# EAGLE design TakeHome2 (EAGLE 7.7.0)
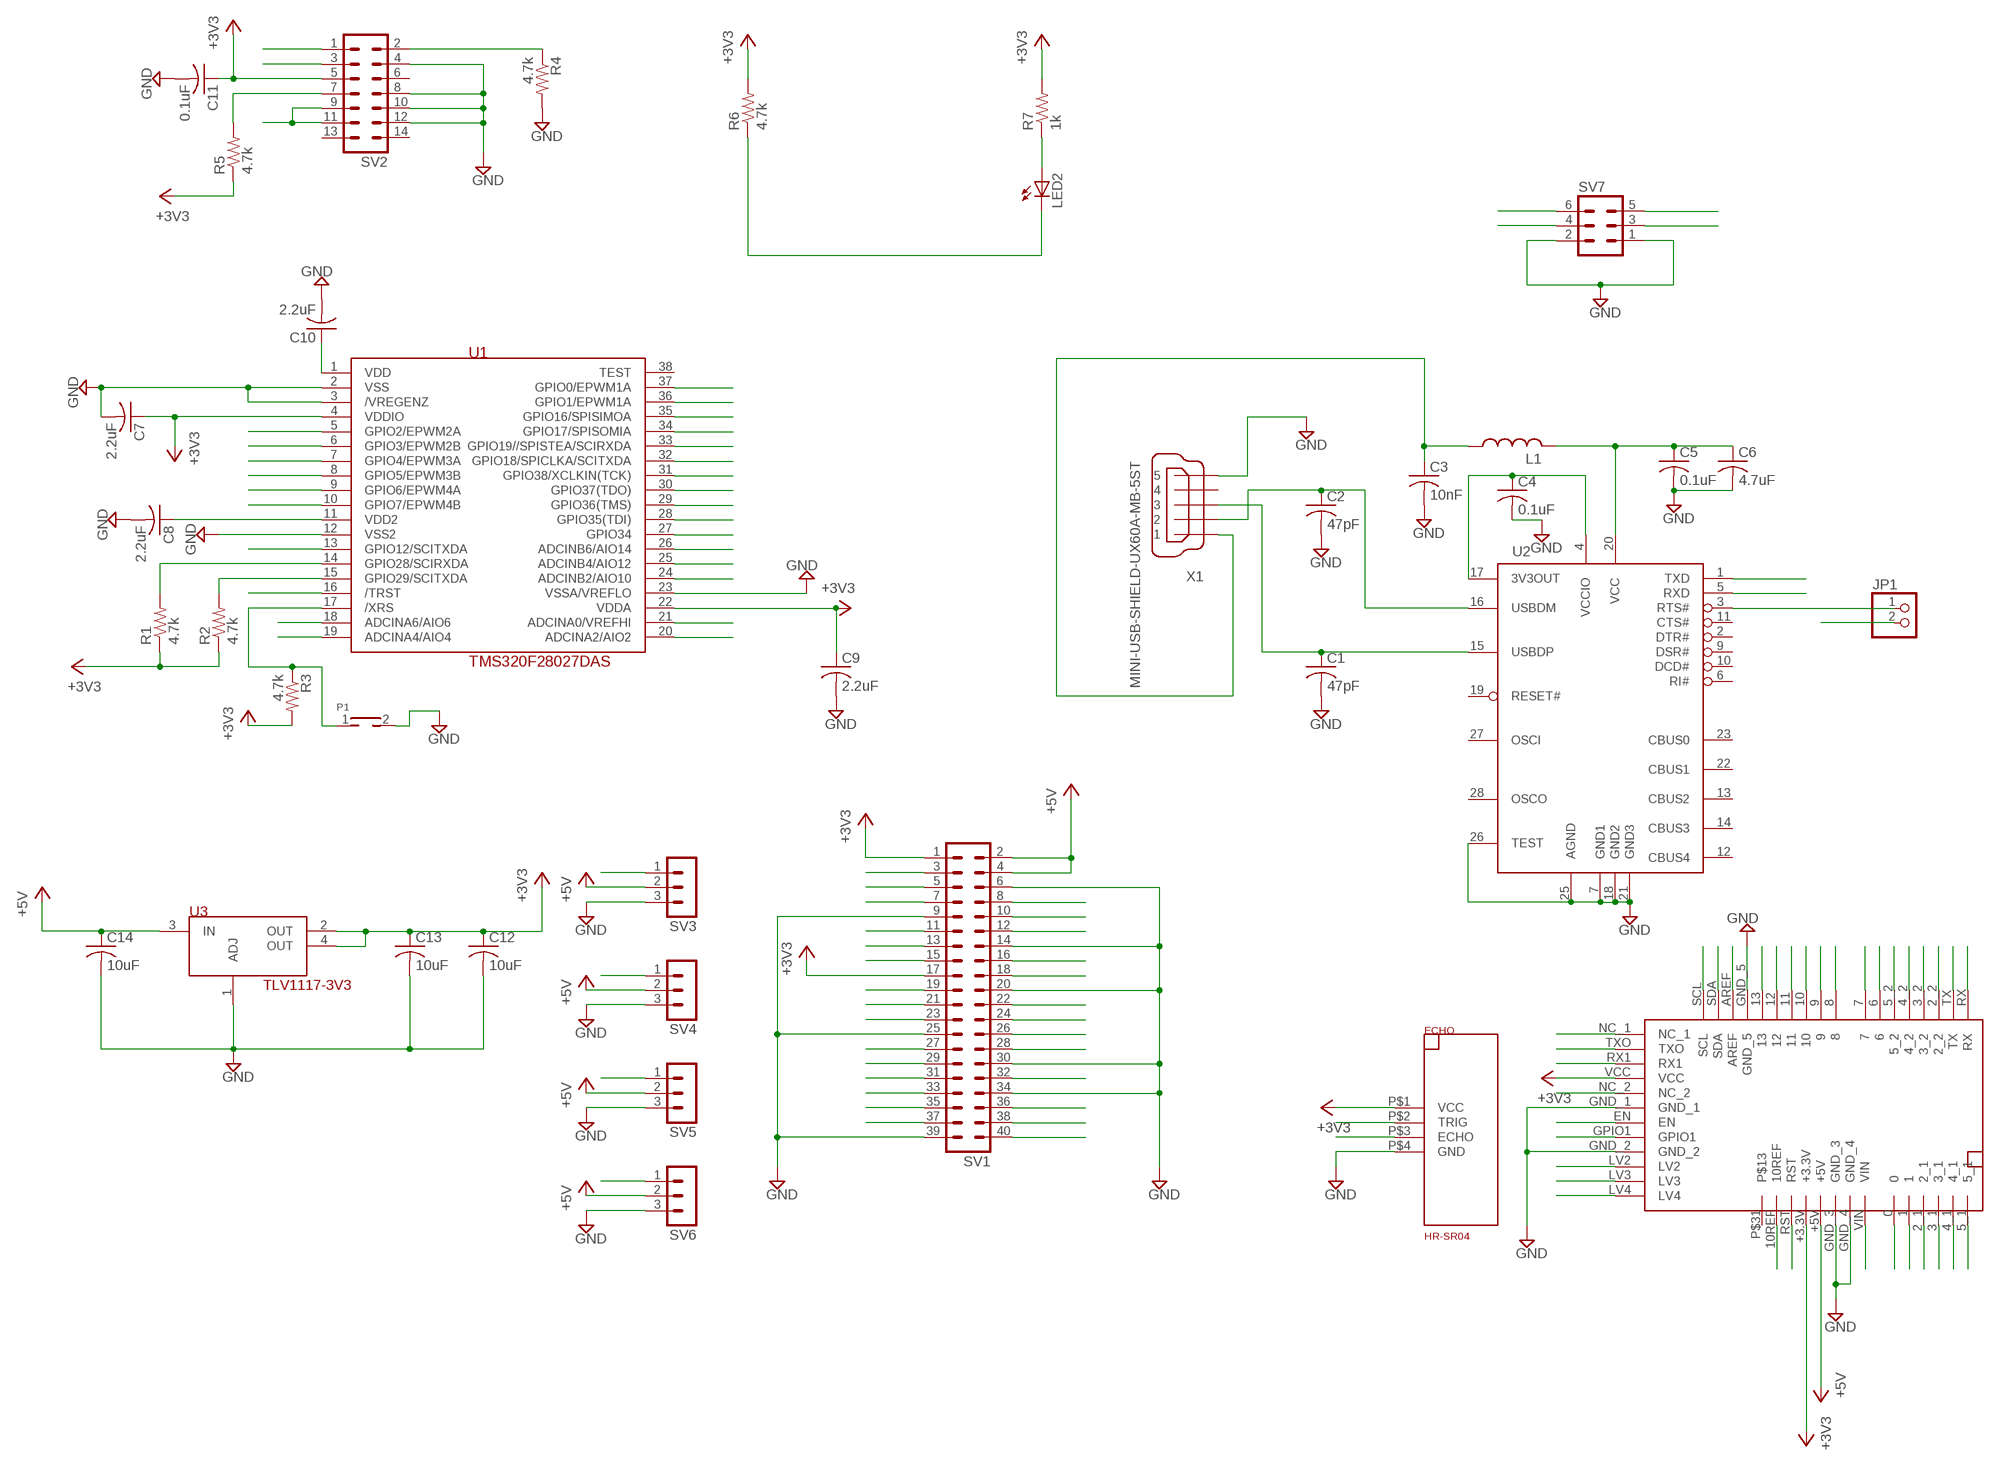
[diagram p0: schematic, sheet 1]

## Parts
C1  47pF  C-US025-025X050  [C025-025X050]
C2  47pF  C-US025-025X050  [C025-025X050]
C3  10nF  C-US025-025X050  [C025-025X050]
C4  0.1uF  C-US025-025X050  [C025-025X050]
C5  0.1uF  C-US025-025X050  [C025-025X050]
C6  4.7uF  C-US025-025X050  [C025-025X050]
C7  2.2uF  C-US025-025X050  [C025-025X050]
C8  2.2uF  C-US025-025X050  [C025-025X050]
C9  2.2uF  C-US025-025X050  [C025-025X050]
C10  2.2uF  C-US025-025X050  [C025-025X050]
C11  0.1uF  C-US025-025X050  [C025-025X050]
C12  10uF  C-US025-025X050  [C025-025X050]
C13  10uF  C-US025-025X050  [C025-025X050]
C14  10uF  C-US025-025X050  [C025-025X050]
ECHO  HR-SR04  [HC-SR04]
JP1  PINHD-1X2  [1X02]
L1  L-US0204/7  [0204/7]
LED2  LED5MM  [LED5MM]
P1  TH_PUSHBOTTON  [TH_PUSHBUTTON]
R1  4.7k  R-US_0204/5  [0204/5]
R2  4.7k  R-US_0204/5  [0204/5]
R3  4.7k  R-US_0204/5  [0204/5]
R4  4.7k  R-US_0204/5  [0204/5]
R5  4.7k  R-US_0204/5  [0204/5]
R6  4.7k  R-US_0204/5  [0204/5]
R7  1k  R-US_0204/5  [0204/5]
SV1  MA20-2  [MA20-2]
SV2  MA07-2  [MA07-2]
SV3  MA03-1  [MA03-1]
SV4  MA03-1  [MA03-1]
SV5  MA03-1  [MA03-1]
SV6  MA03-1  [MA03-1]
SV7  MA03-2  [MA03-2]
U1  TMS320F28027DAS  [DA38]
U2  FT232RL  [SSOP28DB]
U3  TLV1117-3V3  [SOT223]
U$1  M6E_NANO  [M6E_NANO]
X1  MINI-USB-SHIELD-UX60A-MB-5ST  [UX60A-MB-5ST]

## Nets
0: U$1.0
1: U$1.1
2: U$1.2_1 U$1.2_2
3: U$1.3_1 U$1.3_2
4: U$1.4_1 U$1.4_2
5: U$1.5_1 U$1.5_2
6: U$1.6
7: U$1.7
8: U$1.8
9: U$1.9
10: U$1.10
10REF: U$1.10REF
11: U$1.11
12: U$1.12
13: U$1.13
+3V3 [supply]: C7.1 C9.1 C11.1 C12.1 C13.1 ECHO.P$1(VCC) R1.1 R2.1 R3.2 R5.1 R6.2 R7.2 SV1.1 SV1.17 SV2.5 U1.4(VDDIO) U1.22(VDDA) U3.2(OUT) U3.4(OUT) U$1.+3.3V U$1.VCC
+5V [supply]: C14.1 SV1.2 SV1.4 SV3.2 SV4.2 SV5.2 SV6.2 U3.3(IN) U$1.+5V
/SPISTEA: SV1.24 U1.33(GPIO19//SPISTEA/SCIRXDA)
ADCA0: SV1.27 U1.21(ADCINA0/VREFHI)
ADCA2: SV1.29 U1.20(ADCINA2/AIO2)
ADCA4: SV1.31 U1.19(ADCINA4/AIO4)
ADCA6: SV1.33 U1.18(ADCINA6/AIO6)
ADCB2: SV1.26 U1.24(ADCINB2/AIO10)
ADCB4: SV1.28 U1.25(ADCINB4/AIO12)
ADCB6: SV1.32 U1.26(ADCINB6/AIO14)
AREF: U$1.AREF
ECHO: ECHO.P$3(ECHO)
EN: U$1.EN
GND [supply]: C1.2 C2.2 C3.2 C4.2 C5.2 C6.2 C7.2 C8.2 C9.2 C10.2 C11.2 C12.2 C13.2 C14.2 ECHO.P$4(GND) P1.2 R4.2 SV1.6 SV1.9 SV1.14 SV1.20 SV1.25 SV1.30 SV1.34 SV1.39 SV2.4 SV2.8 SV2.10 SV2.12 SV3.3 SV4.3 SV5.3 SV6.3 SV7.1 SV7.2 U1.2(VSS) U1.3(/VREGENZ) U1.12(VSS2) U1.23(VSSA/VREFLO) U2.7(GND1) U2.18(GND2) U2.21(GND3) U2.25(AGND) U2.26(TEST) U3.1(ADJ) U$1.GND_1 U$1.GND_2 U$1.GND_3 U$1.GND_4 U$1.GND_5 X1.5
GPIO0: SV1.7 U1.37(GPIO0/EPWM1A)
GPIO1: SV1.11 U1.36(GPIO1/EPWM1A) U$1.GPIO1
GPIO2: SV1.13 SV3.1 U1.5(GPIO2/EPWM2A)
GPIO3: SV1.15 SV4.1 U1.6(GPIO3/EPWM2B)
GPIO4: SV1.12 SV5.1 U1.7(GPIO4/EPWM3A)
GPIO5: SV1.16 SV6.1 U1.8(GPIO5/EPWM3B)
GPIO6: SV1.18 U1.9(GPIO6/EPWM4A)
GPIO7: SV1.38 U1.10(GPIO7/EPWM4B)
GPIO12: SV1.36 U1.13(GPIO12/SCITXDA)
GPIO34: LED2.K(C) R6.1 SV1.22 U1.27(GPIO34)
LV2: U$1.LV2
LV3: U$1.LV3
LV4: U$1.LV4
N$1: C5.1 C6.1 L1.2 U2.20(VCC)
N$2: C4.1 U2.4(VCCIO) U2.17(3V3OUT)
N$3: C3.1 L1.1 X1.1
N$4: C2.1 U2.16(USBDM) X1.2
N$5: C1.1 U2.15(USBDP) X1.3
N$6: LED2.A R7.1
N$7: C8.1 U1.11(VDD2)
N$8: P1.1 R3.1 U1.17(/XRS)
N$10: C10.1 U1.1(VDD)
N$38: U$1.TX
N$39: U$1.RX
NC: U$1.NC_1 U$1.NC_2
RST: U$1.RST
RTS_FT232RL: JP1.1 U2.3(RTS#)
RX1: U$1.RX1
RXD_FT232RL: SV7.3 U2.5(RXD)
SCL: R2.2 SV1.5 SV1.8 SV7.4 U1.15(GPIO29/SCITXDA) U$1.SCL
SDA: R1.2 SV1.3 SV1.10 SV7.6 U1.14(GPIO28/SCIRXDA) U$1.SDA
SPICLKA: SV1.23 U1.32(GPIO18/SPICLKA/SCITXDA)
SPISIMOA: SV1.19 U1.35(GPIO16/SPISIMOA)
SPISOMIA: SV1.21 U1.34(GPIO17/SPISOMIA)
TCK: SV1.40 SV2.9 SV2.11 U1.31(GPIO38/XCLKIN(TCK))
TDI: SV1.35 SV2.3 U1.28(GPIO35(TDI))
TDO: JP1.2 R5.2 SV2.7 U1.30(GPIO37(TDO))
TMS: SV1.37 SV2.1 U1.29(GPIO36(TMS))
TRIG: ECHO.P$2(TRIG)
TRSTN: R4.1 SV2.2 U1.16(/TRST)
TXD_FT232RL: SV7.5 U2.1(TXD)
TXO: U$1.TXO
VIN: U$1.VIN
Unconnected: SV2.6 SV2.13 SV2.14 U1.38(TEST) U2.2(DTR#) U2.6(RI#) U2.9(DSR#) U2.10(DCD#) U2.11(CTS#) U2.12(CBUS4) U2.13(CBUS2) U2.14(CBUS3) U2.19(RESET#) U2.22(CBUS1) U2.23(CBUS0) U2.27(OSCI) U2.28(OSCO) U$1.P$31 X1.4 X1.M1(S1) X1.M2(S2) X1.M3(S3) X1.M4(S4)

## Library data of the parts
C1-C14 = rcl:C-US: CAPACITOR, American symbol
ECHO = SE423EagleLibrary:HR-SR04
JP1 = pinhead:PINHD-1X2: PIN HEADER
L1 = rcl:L-US: INDUCTOR, American symbol
LED2 = led:LED: LED
P1 = SE423EagleLibrary:TH_PUSHBOTTON
R1-R7 = rcl:R-US_: RESISTOR, American symbol
SV1 = con-lstb:MA20-2: PIN HEADER; OC_FARNELL: unknown; OC_NEWARK: unknown
SV2 = con-lstb:MA07-2: PIN HEADER; OC_FARNELL: unknown; OC_NEWARK: unknown
SV3-SV6 = con-lstb:MA03-1: PIN HEADER; OC_FARNELL: unknown; OC_NEWARK: unknown
SV7 = con-lstb:MA03-2: PIN HEADER; OC_FARNELL: unknown; OC_NEWARK: unknown
U1 = SE423EagleLibrary:TMS320F28027DAS
U2 = SE423EagleLibrary:FT232RL: USB UART 4th Generation USB UART (USB <-> Serial) Controller
U3 = SE423EagleLibrary:TLV1117-3V3
U$1 = SE423EagleLibrary:M6E_NANO
X1 = SE423EagleLibrary:MINI-USB-SHIELD-: MINI USB Connector Source: http://www.hirose.co.jp/cataloge_hp/e24000019.pdf; OC_FARNELL: unknown; OC_NEWARK: unknown

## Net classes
0 default: width 0.203 mm, drill 0.508 mm, clearance 0.203 mm
1 supply: width 0.508 mm, drill 0.508 mm, clearance 0.203 mm

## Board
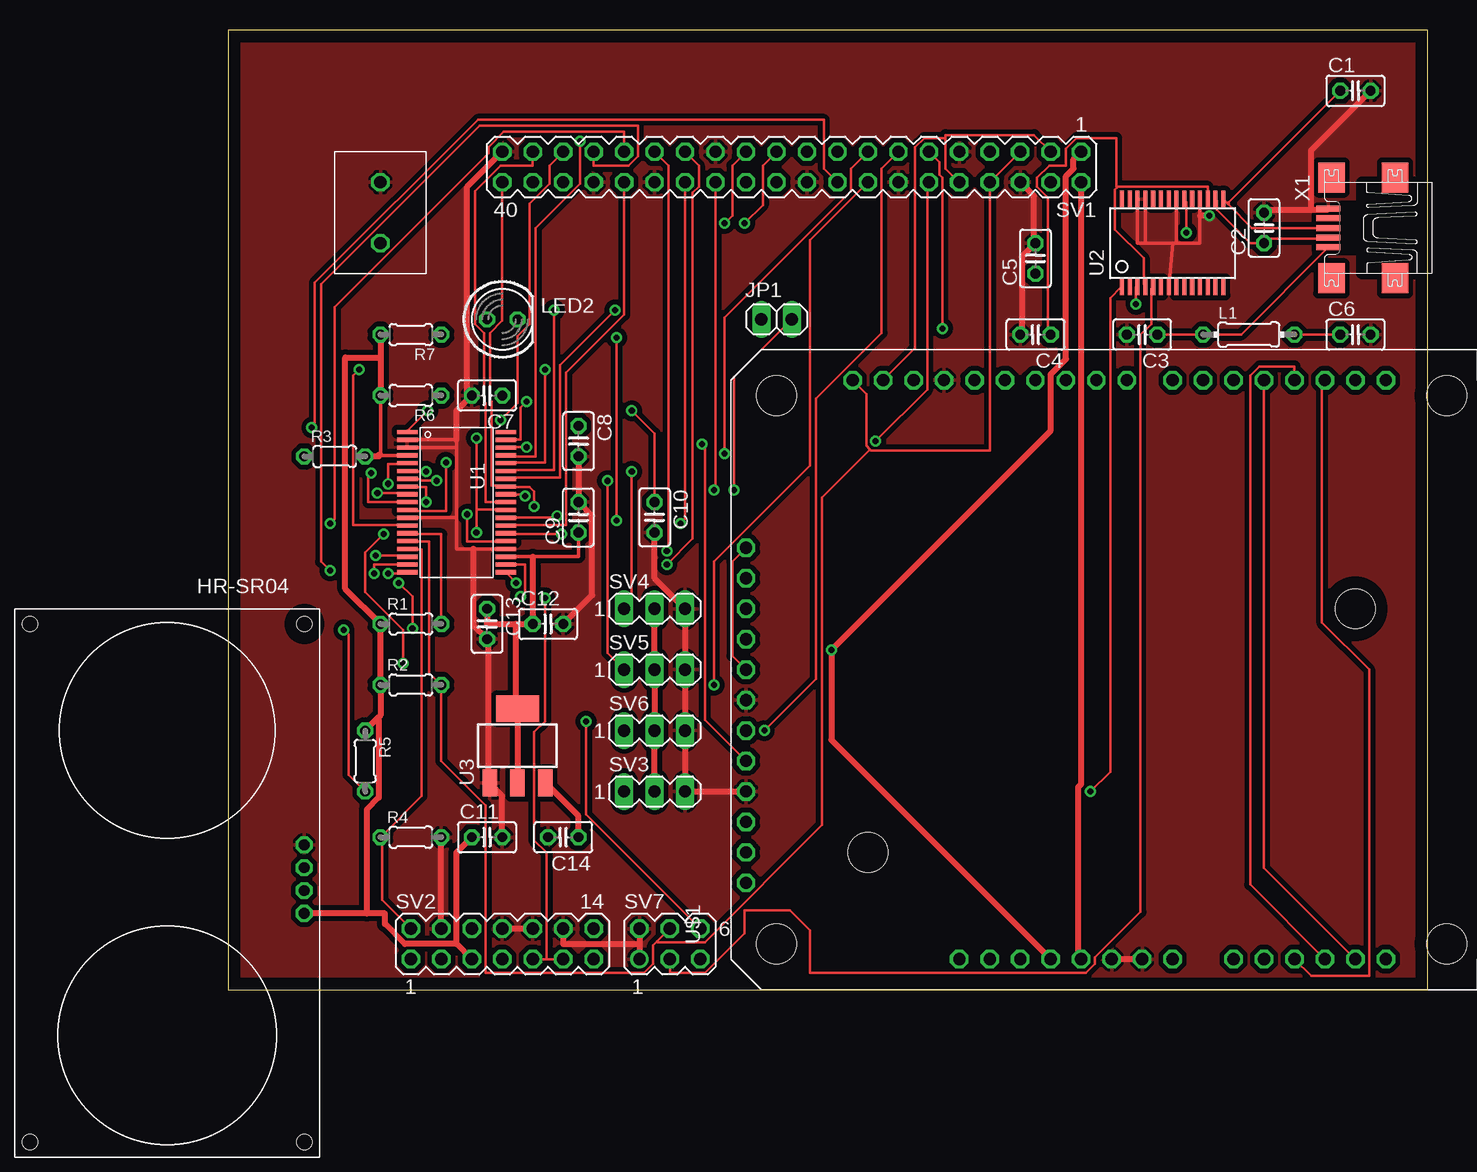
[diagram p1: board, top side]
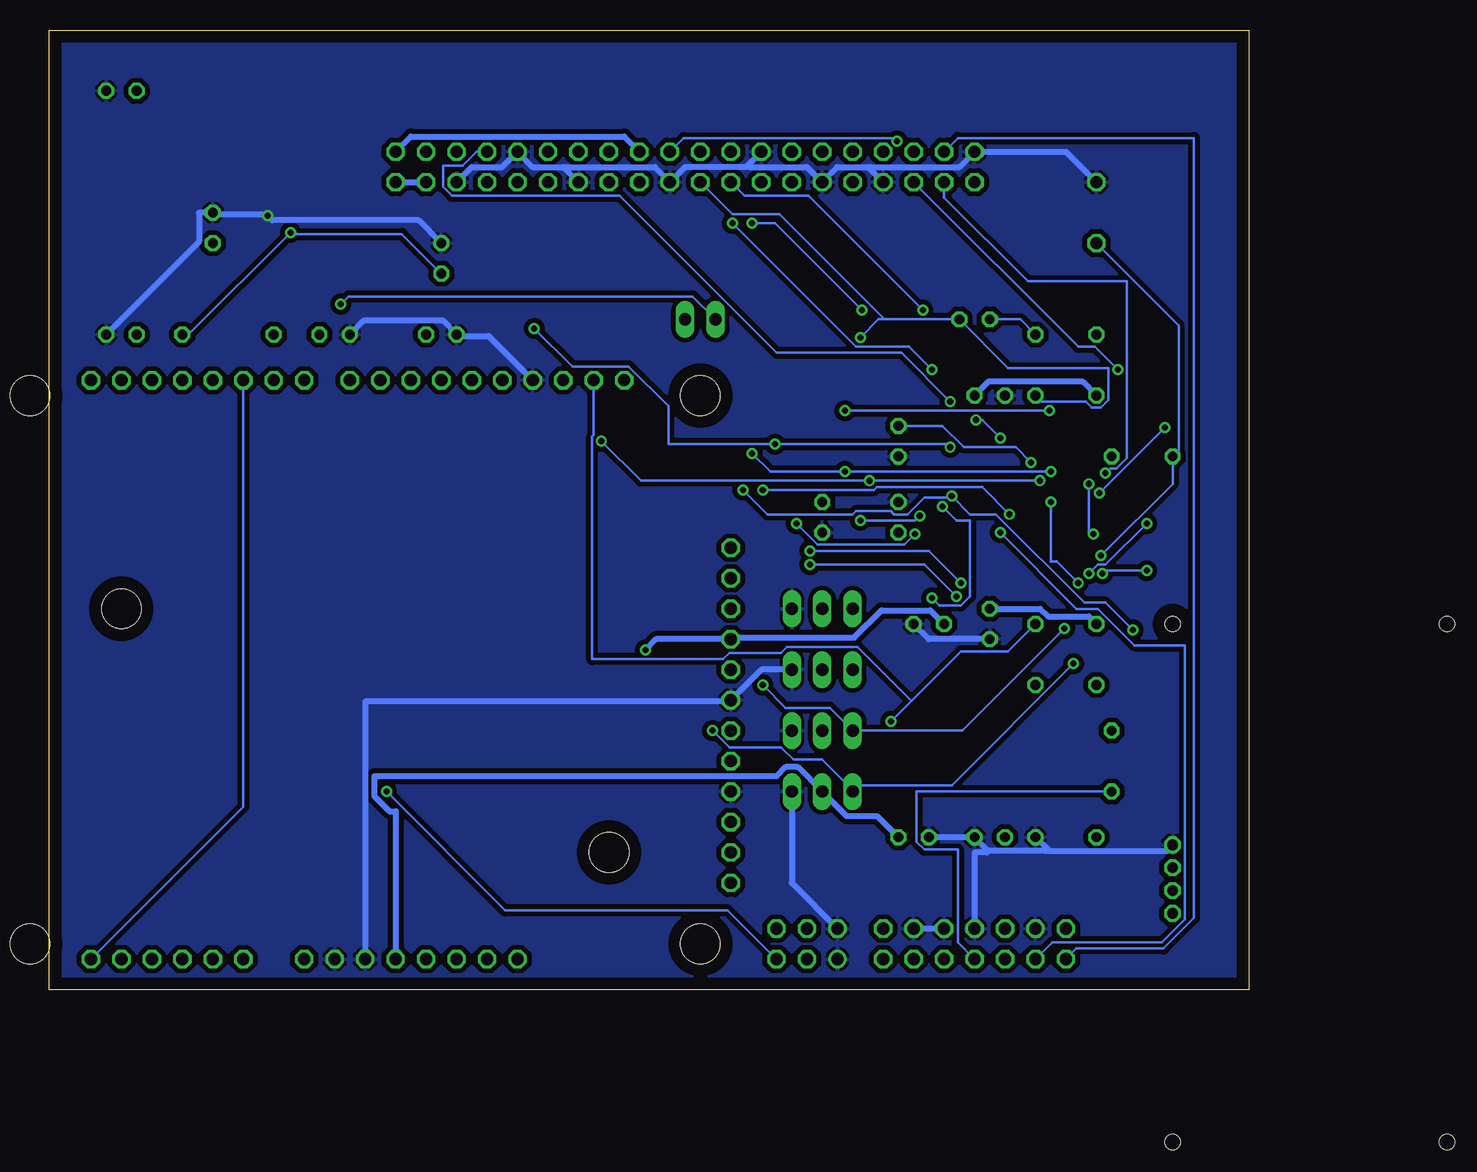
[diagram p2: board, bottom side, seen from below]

Size 100 x 80 mm. Coordinates in mm from the lower left corner, seen from the top.
Outline: 0,0 100,0 100,80 0,80 0,0
Copper layers (1*16): Top 0.035mm / dielectric 1.5mm / Bottom 0.035mm
Design rules "default *": minimum track width 8mil, minimum drill 20mil, track to track 8mil, track to pad 8mil, pad to pad 8mil, via to via 8mil, smd to smd 8mil, copper to edge 40mil, drill to drill 8mil, minimum pad ring 10mil, minimum via ring 8mil, stop-mask expansion 4mil, vias tented up to drill 20mil, thermal gap 10mil

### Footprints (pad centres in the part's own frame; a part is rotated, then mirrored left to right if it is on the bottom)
C025-025X050 = drill 0.813 octagon: 1 -1.27,0; 2 1.27,0
HC-SR04 = drill 0.889 octagon: P$1 1.27,25.4; P$2 1.27,23.495; P$3 1.27,21.59; P$4 1.27,19.685 | hole 1.27: 1.27,1.27; 1.27,44.45; 24.13,44.45; 24.13,1.27
1X02 = drill 1.016 long: 1 -1.27,0; 2 1.27,0
0204/7 = drill 0.813 octagon: 1 -3.81,0; 2 3.81,0
LED5MM = drill 0.813 octagon: A -1.27,0; K 1.27,0
TH_PUSHBUTTON = drill 1.016 octagon: 1 0,2.54; 2 0,-2.54
0204/5 = drill 0.813 octagon: 1 -2.54,0; 2 2.54,0
MA20-2 = drill 1.016 octagon: 1 -24.13,-1.27; 2 -24.13,1.27; 3 -21.59,-1.27; 4 -21.59,1.27; 5 -19.05,-1.27; 6 -19.05,1.27; 7 -16.51,-1.27; 8 -16.51,1.27; 9 -13.97,-1.27; 10 -13.97,1.27; 11 -11.43,-1.27; 12 -11.43,1.27; 13 -8.89,-1.27; 14 -8.89,1.27; 15 -6.35,-1.27; 16 -6.35,1.27; 17 -3.81,-1.27; 18 -3.81,1.27; 19 -1.27,-1.27; 20 -1.27,1.27; 21 1.27,-1.27; 22 1.27,1.27; 23 3.81,-1.27; 24 3.81,1.27; 25 6.35,-1.27; 26 6.35,1.27; 27 8.89,-1.27; 28 8.89,1.27; 29 11.43,-1.27; 30 11.43,1.27; 31 13.97,-1.27; 32 13.97,1.27; 33 16.51,-1.27; 34 16.51,1.27; 35 19.05,-1.27; 36 19.05,1.27; 37 21.59,-1.27; 38 21.59,1.27; 39 24.13,-1.27; 40 24.13,1.27
MA07-2 = drill 1.016 octagon: 1 -7.62,-1.27; 2 -7.62,1.27; 3 -5.08,-1.27; 4 -5.08,1.27; 5 -2.54,-1.27; 6 -2.54,1.27; 7 0,-1.27; 8 0,1.27; 9 2.54,-1.27; 10 2.54,1.27; 11 5.08,-1.27; 12 5.08,1.27; 13 7.62,-1.27; 14 7.62,1.27
MA03-1 = drill 1.016 long: 1 -2.54,0; 2 0,0; 3 2.54,0
MA03-2 = drill 1.016: 1 -2.54,-1.27 | drill 1.016 octagon: 2 -2.54,1.27; 3 0,-1.27; 4 0,1.27; 5 2.54,-1.27; 6 2.54,1.27
DA38 = smd 0.35 x 1.705: 1 -5.85,-4.12; 2 -5.2,-4.12; 3 -4.55,-4.12; 4 -3.9,-4.12; 5 -3.25,-4.12; 6 -2.6,-4.12; 7 -1.95,-4.12; 8 -1.3,-4.12; 9 -0.65,-4.12; 10 0,-4.12; 11 0.65,-4.12; 12 1.3,-4.12; 13 1.95,-4.12; 14 2.6,-4.12; 15 3.25,-4.12; 16 3.9,-4.12; 17 4.55,-4.12; 18 5.2,-4.12; 19 5.85,-4.12; 20 5.85,4.12; 21 5.2,4.12; 22 4.55,4.12; 23 3.9,4.12; 24 3.25,4.12; 25 2.6,4.12; 26 1.95,4.12; 27 1.3,4.12; 28 0.65,4.12; 29 0,4.12; 30 -0.65,4.12; 31 -1.3,4.12; 32 -1.95,4.12; 33 -2.6,4.12; 34 -3.25,4.12; 35 -3.9,4.12; 36 -4.55,4.12; 37 -5.2,4.12; 38 -5.85,4.12
SSOP28DB = smd 0.348 x 1.397: 1 -4.225,-3.656; 2 -3.575,-3.656; 3 -2.925,-3.656; 4 -2.275,-3.656; 5 -1.625,-3.656; 6 -0.975,-3.656; 7 -0.325,-3.656; 8 0.325,-3.656; 9 0.975,-3.656; 10 1.625,-3.656; 11 2.275,-3.656; 12 2.925,-3.656; 13 3.575,-3.656; 14 4.225,-3.656; 15 4.225,3.656; 16 3.575,3.656; 17 2.925,3.656; 18 2.275,3.656; 19 1.625,3.656; 20 0.975,3.656; 21 0.325,3.656; 22 -0.325,3.656; 23 -0.975,3.656; 24 -1.625,3.656; 25 -2.275,3.656; 26 -2.925,3.656; 27 -3.575,3.656; 28 -4.225,3.656
SOT223 = smd 1.219 x 2.235: 1 -2.311,-3.099; 2 0,-3.099; 3 2.311,-3.099 | smd 3.6 x 2.2: 4 0,3.099
M6E_NANO = drill 1.016 octagon: 0 41.91,2.54; 1 44.45,2.54; 2_1 46.99,2.54; 2_2 49.53,50.8; 3_1 49.53,2.54; 3_2 46.99,50.8; 4_1 52.07,2.54; 4_2 44.45,50.8; 5_1 54.61,2.54; 5_2 41.91,50.8; 6 39.37,50.8; 7 36.83,50.8; 8 33.02,50.8; 9 30.48,50.8; 10 27.94,50.8; 10REF 21.59,2.54; 11 25.4,50.8; 12 22.86,50.8; 13 20.32,50.8; +3.3V 26.67,2.54; +5V 29.21,2.54; AREF 15.24,50.8; EN 1.27,21.59; GND_1 1.27,24.13; GND_2 1.27,16.51; GND_3 31.75,2.54; GND_4 34.29,2.54; GND_5 17.78,50.8; GPIO1 1.27,19.05; LV2 1.27,13.97; LV3 1.27,11.43; LV4 1.27,8.89; NC_1 1.27,36.83; NC_2 1.27,26.67; P$31 19.05,2.54; RST 24.13,2.54; RX 54.61,50.8; RX1 1.27,31.75; SCL 10.16,50.8; SDA 12.7,50.8; TX 52.07,50.8; TXO 1.27,34.29; VCC 1.27,29.21; VIN 36.83,2.54 | hole 3.302: 3.81,3.81; 11.43,11.43; 3.81,49.53; 59.69,49.53; 59.69,3.81; 52.07,31.75
UX60A-MB-5ST = smd 2 x 0.5: 1 2.25,1.6; 2 2.25,0.8; 3 2.25,0; 4 2.25,-0.8; 5 2.25,-1.6 | smd 2.2 x 2.5: M1 -3.3,-4.2; M2 -3.3,4.2; M3 2,4.2; M4 2,-4.2

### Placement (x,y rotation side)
C1  93.98,74.93 0 top
C2  86.36,63.5 90 top
C3  76.2,54.61 180 top
C4  67.31,54.61 180 top
C5  67.31,60.96 90 top
C6  93.98,54.61 0 top
C7  21.59,49.53 180 top
C8  29.21,45.72 270 top
C9  29.21,39.37 90 top
C10  35.56,39.37 270 top
C11  21.59,12.7 0 top
C12  26.67,30.48 0 top
C13  21.59,30.48 270 top
C14  27.94,12.7 180 top
ECHO  7.62,31.75 180 top
JP1  45.72,55.88 0 top
L1  85.09,54.61 0 top
LED2  22.86,55.88 0 top
P1  12.7,64.77 180 top
R1  15.24,30.48 0 top
R2  15.24,25.4 0 top
R3  8.89,44.45 0 top
R4  15.24,12.7 0 top
R5  11.43,19.05 270 top
R6  15.24,49.53 180 top
R7  15.24,54.61 180 top
SV1  46.99,68.58 180 top
SV2  22.86,3.81 0 top
SV3  35.56,16.51 0 top
SV4  35.56,31.75 0 top
SV5  35.56,26.67 0 top
SV6  35.56,21.59 0 top
SV7  36.83,3.81 0 top
U1  19.05,40.64 270 top
U2  78.74,62.23 0 top
U3  24.13,20.32 0 top
U$1  41.91,0 0 top
X1  93.98,63.5 180 top

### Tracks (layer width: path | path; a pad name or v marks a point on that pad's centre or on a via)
2
  Top 0.203: U$1.2_1 90.3,1.14 95.12,1.14 95.12,26.67 91.19,30.61 91.19,50.55 U$1.2_2
3
  Top 0.203: U$1.3_1 85.22,8.76 85.22,51.18 85.98,51.94 88.9,51.94 U$1.3_2
4
  Top 0.203: U$1.4_1 86.36,10.16 U$1.4_2
5
  Bottom 0.203: U$1.5_1 83.82,15.24 U$1.5_2
+3V3  (via drill 0.51)
  Top 0.305: U1.22 25.4,36.09 29.21,36.09 C9.1 | U1.4 12.7,44.54 12.7,44.58 R6.2
  Top 0.508: C11.1 19.05,11.43 19.05,3.81 | SV2.5 19.05,3.81 | 11.56,6.35 13.08,6.35 13.08,5.46 14.73,3.81 19.05,3.81 | 11.56,6.35 ECHO.P$1 | R3.2 12.57,44.45 12.57,44.58 12.7,44.58 | R7.2 12.7,52.7 | 12.7,52.7 R6.2 | 12.45,22.61 12.7,22.86 R2.1 R1.1 9.78,33.4 9.78,52.7 12.7,52.7 | 12.45,22.61 R5.1 | 24,30.48 21.59,30.48 C13.1 | 24,30.48 C12.1 25.4,36.09 | U3.2 U3.4 24,23.62 24,30.48 | 11.56,6.35 11.56,14.99 12.57,16 12.57,22.48 12.45,22.61 | U$1.+3.3V 50.29,20.83 v50.29,28.32 68.58,46.61 68.58,51.31 69.85,52.58 69.85,67.82 70.48,68.45 70.48,69.22 SV1.1
  Bottom 0.508: C7.1 21.72,50.67 13.84,50.67 R6.2 | R1.1 13.34,31.11 16.76,31.11 17.4,31.75 C13.1 | SV1.17 52.07,71.12 69.85,71.12 SV1.1 | v50.29,28.32 49.4,29.21 U$1.VCC 43.05,29.34 32.89,29.34 30.61,31.62 26.54,31.62 C12.1
+5V
  Top 0.508: SV4.2 SV5.2 SV6.2 SV3.2 | C14.1 29.21,14.48 26.54,17.14 U3.3 | SV1.2 71.12,17.14 70.87,16.89 70.87,2.79 U$1.+5V
  Bottom 0.508: SV1.2 SV1.4 | U$1.+5V 71.12,14.86 71.63,14.86 72.9,16.13 72.9,17.78 39.37,17.78 38.61,18.54 37.59,18.54 SV3.2 33.53,14.48 30.99,14.48 C14.1
/SPISTEA  (via drill 0.51)
  Top 0.203: v27.18,56.64 27.18,43.31 23.24,43.31 U1.33
  Bottom 0.203: v27.18,56.64 36.7,66.17 42.04,66.17 SV1.24
ADCA0  (via drill 0.51)
  Top 0.203: v24.38,32.77 24.77,33.15 24.77,35.43 23.24,35.43 U1.21 | v36.58,35.43 38.73,37.59 38.73,66.42 39.24,66.93 39.24,68.71 SV1.27
  Bottom 0.203: v24.38,32.77 27.05,35.43 v36.58,35.43
ADCA2  (via drill 0.51)
  Top 0.203: v24,33.91 23.24,34.67 U1.20 | v36.58,36.58 36.7,36.7 36.7,68.71 SV1.29
  Bottom 0.203: v24,33.91 26.67,36.58 v36.58,36.58
ADCA4  (via drill 0.51)
  Top 0.203: v13.34,34.67 14.86,34.67 U1.19 | v8.51,38.86 8.89,39.24 8.89,56.9 21.72,69.72 21.72,70.23 22.99,71.5 33.02,71.5 SV1.31
  Bottom 0.203: v13.34,34.67 12.57,35.43 11.94,35.43 v8.51,38.86
ADCA6  (via drill 0.51)
  Top 0.203: v12.19,34.67 12.19,35.43 14.86,35.43 U1.18 | v8.51,34.92 7.75,35.69 7.75,58.8 20.95,72.01 34.16,72.01 34.16,69.47 33.4,68.71 30.48,68.71 SV1.33
  Bottom 0.203: v12.19,34.67 11.94,34.92 v8.51,34.92
ADCB2  (via drill 0.51)
  Top 0.203: v19.94,39.62 19.94,37.34 23.11,37.34 U1.24 | v40.51,41.66 40.64,41.78 SV1.26
  Bottom 0.203: v19.94,39.62 22.23,41.91 30.99,41.91 31.24,41.66 v40.51,41.66
ADCB4  (via drill 0.51)
  Top 0.203: v27.81,37.97 23.24,37.97 U1.25 | v37.72,38.86 38.1,39.24 SV1.28
  Bottom 0.203: v27.81,37.97 28.7,37.08 35.94,37.08 v37.72,38.86
ADCB6
  Top 0.203: SV1.32 33.02,56.26 28.19,51.44 28.19,38.73 23.24,38.73 U1.26
GND  (via drill 0.51)
  Top 0.305: U1.23 20.45,36.74 19.05,36.74 19.05,39.34 | U1.12 19.05,39.34 | U1.2 19.05,45.84 19.05,45.19 | 19.05,45.19 19.05,39.34 | U1.3 19.05,45.19 | U2.7 78.74,62.23 | 78.74,62.23 76.47,62.23 | 76.47,62.23 75.81,62.23 U2.26 | U2.25 76.47,62.23 | U2.21 79.06,62.23 | 79.06,62.23 78.74,62.23 | U2.18 81.02,64.52 81.02,62.23 79.06,62.23
  Top 0.508: 90.3,65.02 86.36,65.02 C2.2 | 90.3,65.02 91.69,65.02 X1.5 | C1.2 90.3,69.98 90.3,65.02 | v81.79,64.52 81.02,64.52 | C4.2 66.17,54.74 66.17,61.09 C5.2 67.18,62.36 67.18,66.17 SV1.6 | C8.2 C9.2 30.35,39.5 30.35,32.89 C12.2 | 20.45,36.74 20.45,30.35 C13.2 21.72,29.08 21.72,17.4 U3.1 21.84,17.14 22.86,16.13 C11.2 | 19.05,45.84 19.05,48.26 C7.2 19.94,49.4 19.94,66.93 SV1.39 | SV7.2 34.29,3.81 | 34.29,3.81 SV7.1 | SV2.10 SV2.8 | 34.29,3.81 27.94,3.81 SV2.12 | SV2.4 R4.2 | U$1.GND_2 SV3.3 SV6.3 SV5.3 SV4.3 35.56,34.29 C10.2 | U$1.GND_4 U$1.GND_3
  Bottom 0.508: P1.2 15.24,69.85 SV1.39 24.13,68.58 31.5,68.58 31.62,68.45 | 31.62,68.45 31.75,68.58 34.29,68.58 SV1.30 36.83,68.58 41.66,68.58 41.78,68.71 | 31.62,68.45 SV1.34 | SV1.25 41.78,68.71 | 41.78,68.71 41.91,68.58 46.99,68.58 SV1.20 49.53,68.58 56.9,68.58 57.02,68.45 | C6.2 87.5,62.36 87.5,64.77 C2.2 86.23,64.64 81.92,64.64 v81.79,64.52 81.41,64.14 69.22,64.14 C5.2 | 57.02,68.45 57.15,68.58 59.69,68.58 SV1.9 62.23,68.58 64.77,68.58 SV1.6 | 57.02,68.45 SV1.14 | C3.2 73.79,55.75 67.18,55.75 C4.2 65.91,54.48 63.37,54.48 U$1.GND_5 | C12.2 26.67,29.21 C13.2 | SV2.10 SV2.12 | C14.2 C11.2 21.72,11.56 | ECHO.P$4 6.86,11.56 16.64,11.56 16.76,11.68 | R4.2 16.76,11.68 | 21.72,11.56 16.89,11.56 16.76,11.68 | SV2.8 22.86,11.43 21.84,11.43 21.72,11.56 | SV5.3 40.64,26.67 U$1.GND_1 43.31,24 73.66,24 U$1.GND_3 | SV7.2 38.1,8.89 SV3.3
  pour Top (isolate 0.406): 0,80.01 100.33,80.01 100.33,0 0,0
  pour Bottom (isolate 0.406): 0,80.01 100.33,80.01 100.33,0 0,0
GPIO0  (via drill 0.51)
  Top 0.203: v24.89,49.02 24.38,48.51 24.38,45.85 23.24,45.85 U1.37
  Bottom 0.203: v24.89,49.02 28.96,53.09 39.37,53.09 52.45,66.17 66.42,66.17 67.18,66.93 67.18,68.71 65.53,68.71 64.39,69.85 SV1.7
GPIO1  (via drill 0.51)
  Top 0.203: v24.89,45.21 23.24,45.21 U1.36 | v39.5,45.47 39.75,45.21 39.75,22.48 U$1.GPIO1 | SV1.11 59.31,68.96 59.31,67.94 59.56,67.69 v59.56,55.12
  Bottom 0.203: v24.89,45.21 25.15,45.47 v39.5,45.47 48.39,45.47 48.39,48.64 51.69,51.94 56.39,51.94 v59.56,55.12
GPIO2  (via drill 0.51)
  Top 0.203: v13.34,42.16 13.34,43.81 14.86,43.81 U1.5 | v12.95,37.97 11.43,36.45 11.43,33.15 14.61,29.97 v14.61,27.18 | SV1.13 54.48,68.45 54.48,54.74 49.02,49.28 49.02,25.91 v44.7,21.59
  Bottom 0.203: v13.34,42.16 13.34,37.97 v12.95,37.97 | v14.61,27.18 24.77,17.02 32.51,17.02 SV3.1 33.02,16.64 35.56,19.18 37.97,19.18 38.99,20.19 43.31,20.19 v44.7,21.59
GPIO3  (via drill 0.51)
  Top 0.203: v16.51,43.18 14.99,43.18 U1.6 | v33.66,43.18 33.66,32.38 SV4.1 | SV1.15 51.94,68.45 51.94,66.55 41.4,56.01 v41.4,44.7
  Bottom 0.203: v16.51,43.18 v33.66,43.18 39.88,43.18 v41.4,44.7
GPIO4  (via drill 0.51)
  Top 0.203: v17.4,42.42 16.13,42.42 16,42.55 14.99,42.55 U1.7 | v31.62,42.42 31.62,28.07 SV5.1 | SV1.12 58.29,67.18 58.29,50.04 v53.98,45.72
  Bottom 0.203: v17.4,42.42 v31.62,42.42 50.67,42.42 v53.98,45.72
GPIO5  (via drill 0.51)
  Top 0.203: v16.51,40.64 16.51,41.91 14.99,41.91 U1.8 | v14.22,33.91 15.37,32.77 v15.37,30.1 | SV1.16 48.51,62.48 48.51,43.69 40.51,35.69 v40.51,25.4
  Bottom 0.203: v16.51,40.64 16.51,35.69 16,35.69 v14.22,33.91 | v15.37,30.1 23.88,21.59 SV6.1 34.92,23.5 38.61,23.5 v40.51,25.4
GPIO6  (via drill 0.51)
  Top 0.203: v12.45,41.4 14.86,41.4 U1.9 | v6.99,46.86 7.24,47.12 7.24,58.93 20.83,72.52 49.66,72.52 49.66,68.45 SV1.18
  Bottom 0.203: v6.99,46.86 v12.45,41.4
GPIO7  (via drill 0.51)
  Top 0.203: U1.10 11.68,40.64 11.68,42.8 v11.94,43.05
  Bottom 0.203: v11.94,43.05 11.56,43.43 11.05,43.43 10.16,44.32 10.16,59.05 18.41,59.05 25.4,66.04 SV1.38
GPIO12  (via drill 0.51)
  Top 0.203: v10.92,51.69 10.41,51.18 10.41,38.73 14.86,38.73 U1.13
  Bottom 0.203: v10.92,51.69 12.83,53.59 14.22,53.59 SV1.36
GPIO34  (via drill 0.51)
  Top 0.203: v27.43,39.5 27.43,39.37 23.24,39.37 U1.27 | v32.38,54.36 v32.38,39.12
  Bottom 0.203: v27.43,39.5 27.81,39.12 v32.38,39.12 | v32.38,54.36 30.86,55.88 30.35,55.88 | 30.35,55.88 LED2.K 20.07,51.82 11.68,51.82 11.68,49.15 12.32,48.51 13.08,48.51 13.59,49.02 17.27,49.02 R6.1 | SV1.22 43.05,64.64 39.12,64.64 30.35,55.88
N$1  (via drill 0.51)
  Top 0.203: v79.88,63.12 79.88,65.66 79.76,65.79 U2.20 | L1.2 C6.1
  Bottom 0.203: L1.2 88.39,54.61 v79.88,63.12 79.88,62.99 70.61,62.99 C5.1
N$2
  Top 0.203: 74.11,66.86 74.17,66.93 81.66,66.93 81.66,65.91 U2.17 | 74.11,66.86 73.91,66.67 73.91,63.37 76.33,60.96 76.33,58.8 76.45,58.67 U2.4 | C4.1 68.33,54.86 68.33,66.04 67.44,66.93 67.44,67.69 68.45,68.71 69.85,68.71 69.85,70.1 70.74,70.99 74.04,70.99 74.04,66.93 74.11,66.86
N$3
  Top 0.203: X1.1 91.69,61.85 84.45,54.61 L1.1 C3.1
N$4
  Top 0.203: U2.16 82.42,65.79 82.42,65.02 85.22,62.23 C2.1 86.36,62.61 91.69,62.61 X1.2
N$5
  Top 0.203: 83.38,65.47 85.34,63.5 X1.3 | 83.38,65.47 83.06,65.79 U2.15 | C1.1 83.44,65.66 83.44,65.53 83.38,65.47
N$6
  Bottom 0.203: R7.1 19.05,55.88 LED2.A
N$7  (via drill 0.51)
  Top 0.203: v18.16,43.94 18.16,39.88 14.99,39.88 U1.11
  Bottom 0.203: v18.16,43.94 19.43,45.21 23.75,45.21 25.53,46.99 C8.1
N$8  (via drill 0.51)
  Top 0.203: v12.32,36.2 14.86,36.2 U1.17
  Bottom 0.203: v12.32,36.2 6.35,42.16 R3.1 5.84,44.45 5.84,55.37 P1.1
N$10  (via drill 0.51)
  Top 0.203: v16.64,48.26 14.99,46.61 U1.1 | v33.66,48.26 35.56,46.35 C10.1
  Bottom 0.203: v33.66,48.26 v16.64,48.26
NC
  Top 0.203: U$1.NC_2 42.04,27.81 42.04,35.69 U$1.NC_1
RTS_FT232RL  (via drill 0.51)
  Top 0.203: v75.69,57.15 75.69,58.55 U2.3
  Bottom 0.203: v75.69,57.15 75.06,57.78 46.35,57.78 JP1.1
RXD_FT232RL
  Top 0.203: SV7.3 36.83,1.4 39.75,1.4 43.05,4.7 43.05,6.6 46.86,6.6 48.51,4.95 48.51,1.4 71.5,1.4 72.26,2.16 72.26,2.67 76.07,6.48 76.07,54.61 76.96,55.5 76.96,58.42 77.09,58.55 U2.5
SCL
  Top 0.203: U$1.SCL 53.21,49.66 53.21,45.34 53.53,45.02 | 53.53,45.02 53.59,44.96 63.5,44.96 SV1.8 SV1.5 | U1.15 14.99,37.34 16.76,37.34 16.76,26.42 R2.2 17.78,19.05 21.46,15.37 21.46,1.4 34.67,1.4 35.43,2.16 35.43,3.68 35.75,4 | 35.75,4 SV7.4 | 53.53,45.02 49.53,41.02 49.53,13.72 39.75,3.94 35.81,3.94 35.75,4
SDA  (via drill 0.51)
  Top 0.203: U$1.SDA 57.28,53.47 57.28,70.23 58.04,70.99 59.82,70.99 | 59.82,70.99 59.82,68.45 SV1.10 | SV1.3 67.18,71.25 59.82,71.25 59.82,70.99 | R1.2 17.78,37.97 14.99,37.97 U1.14 | SV7.6 29.84,14.61 v29.84,22.35
  Bottom 0.203: 28.13,24.07 24,28.19 20.07,28.19 R1.2 | 28.13,24.07 v29.84,22.35 | U$1.SDA 54.61,46.23 54.74,46.1 54.74,27.56 43.81,27.56 43.31,28.07 38.99,28.07 38.48,28.57 32.64,28.57 28.13,24.07
SPICLKA  (via drill 0.51)
  Top 0.203: v32.26,56.64 27.69,52.07 27.69,42.67 23.24,42.67 U1.32 | v41.4,63.88 42.04,64.52 42.04,68.71 SV1.23
  Bottom 0.203: v32.26,56.64 39.5,63.88 v41.4,63.88
SPISIMOA  (via drill 0.51)
  Top 0.203: v29.34,70.74 29.34,67.18 25.65,63.5 25.65,44.45 23.24,44.45 U1.35
  Bottom 0.203: v29.34,70.74 29.59,70.99 47.12,70.99 SV1.19
SPISOMIA  (via drill 0.51)
  Top 0.203: v26.42,51.69 26.42,43.94 23.24,43.94 U1.34 | v43.05,63.88 44.58,65.41 44.58,68.71 SV1.21
  Bottom 0.203: v26.42,51.69 28.32,53.59 32.77,53.59 v43.05,63.88
TCK  (via drill 0.51)
  Top 0.203: SV2.11 26.54,2.54 | 26.54,2.54 SV2.9 | SV1.40 22.86,55.75 21.84,54.74 21.84,49.15 21.97,49.02 21.97,42.04 23.11,42.04 U1.31 23.24,41.91 25.15,41.91 25.53,41.53 v25.53,40.26 | 26.54,2.54 26.54,11.43 25.53,12.45 25.53,21.46 26.42,22.35 v26.42,32.64
  Bottom 0.203: v26.42,32.64 25.78,32 24,32 23.24,32.77 23.24,39.12 24.38,39.12 v25.53,40.26
TDI  (via drill 0.51)
  Top 0.203: 20.7,40.01 23.11,40.01 U1.28 | v20.7,45.97 20.7,40.01 | v22.73,47.5 24.13,48.9 24.13,54.48 25.15,55.5 25.15,65.53 26.8,67.18 26.8,68.71 SV1.35 | 20.7,40.01 v20.7,38.1
  Bottom 0.203: v20.7,45.97 22.23,47.5 v22.73,47.5 | SV2.3 16.38,3.94 7.24,3.94 5.33,5.84 5.33,28.7 9.53,28.7 12.57,31.75 14.35,31.75 v20.7,38.1
TDO  (via drill 0.51)
  Top 0.203: v24.77,41.15 24.77,41.27 23.24,41.27 U1.30 | v9.65,29.97 10.03,29.59 10.03,17.91 R5.2 | JP1.2 42.16,51.05 v42.16,41.66
  Bottom 0.203: v9.65,29.97 11.94,32.26 13.72,32.26 21.08,39.62 23.24,39.62 v24.77,41.15 24.77,41.02 27.05,41.02 28.45,39.62 29.59,39.62 29.84,39.88 32.77,39.88 33.02,39.62 40.13,39.62 v42.16,41.66 | SV2.7 24.26,3.94 24.26,11.68 27.05,11.68 27.69,12.32 27.69,16.51 R5.2
TMS
  Top 0.203: U1.29 21.46,40.64 21.46,48.9 21.34,49.02 21.34,54.74 20.57,55.5 20.57,66.55 22.73,68.71 25.4,68.71 SV1.37
  Bottom 0.203: SV2.1 14.35,3.43 7.11,3.43 4.57,5.97 4.57,70.99 24.26,70.99 SV1.37
TRSTN
  Top 0.203: U1.16 14.99,36.7 16.13,36.7 16.13,16.13 R4.1 12.83,12.7 12.83,7.49 SV2.2
TXD_FT232RL  (via drill 0.51)
  Top 0.203: v71.88,16.51 73.53,18.16 73.53,57.66 74.42,58.55 U2.1
  Bottom 0.203: v71.88,16.51 61.98,6.6 43.43,6.6 SV7.5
